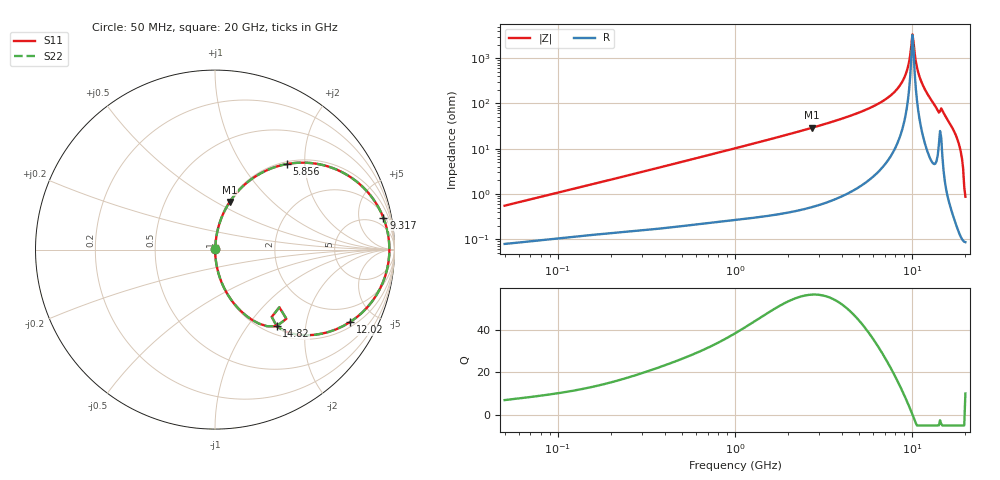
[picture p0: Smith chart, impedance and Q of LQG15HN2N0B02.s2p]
!Murata Part Number: LQG15HN2N0B02
!These Parameters are Measured in Series Mode Connection
!  o--[Z]--o
!Port1  Port2
!  o-------o
!Freq. Start=50[MHz] Stop=20[GHz], 401[Steps]
# Hz S RI R 50
!Freq.(Hz) S11(Real) S11(Imag) S21(Real) S21(Imag) S12(Real) S12(Imag) S22(Real) S22(Imag)
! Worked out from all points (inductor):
!   401 points, 50 MHz to 20 GHz, reference 50 ohm
!   read as one part in series: L = 1.72 nH near 51.52 MHz
!   highest Q = 56.5 at 2.728 GHz (marker M1), where L = 1.69 nH
!   self-resonance near 10.04 GHz
!   S11 on the Smith chart (normalised r, x): 50 MHz: 1.00, +0.01; 5.856 GHz: 1.04, +1.63; 9.317 GHz: 2, +10; 12.02 GHz: 1.21, -3.60; 14.82 GHz: 1.14, -1.39; 20 GHz: 1.00, +0.02
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5e7  0.000816 0.00544  0.9992 -0.00544  0.9992 -0.00544  0.000816 0.00544
1.364002e8  0.00139 0.0143  0.9986 -0.0143  0.9986 -0.0143  0.00139 0.0143
3.721004e8  0.00315 0.038  0.9968 -0.038  0.9968 -0.038  0.00315 0.038
1e9  0.0128 0.1002  0.9872 -0.1002  0.9872 -0.1002  0.0128 0.1002
2.728004e9  0.0817 0.2652  0.9183 -0.2652  0.9183 -0.2652  0.0817 0.2652
4.212059e9  0.1986 0.3892  0.8014 -0.3892  0.8014 -0.3892  0.1986 0.3892
5.856089e9  0.4012 0.4769  0.5988 -0.4769  0.5988 -0.4769  0.4012 0.4769
7.442007e9  0.6629 0.4516  0.3371 -0.4516  0.3371 -0.4516  0.6629 0.4516
8.516016e9  0.8415 0.3307  0.1585 -0.3307  0.1585 -0.3307  0.8415 0.3307
9.316812e9  0.938 0.1778  0.062 -0.1778  0.062 -0.1778  0.938 0.1778
9.892087e9  0.9698 0.0432  0.0302 -0.0432  0.0302 -0.0432  0.9698 0.0432
1.004137e10  0.9716 0.00642  0.0284 -0.00642  0.0284 -0.00642  0.9716 0.00642
1.034674e10  0.9666 -0.0692  0.0334 0.0692  0.0334 0.0692  0.9666 -0.0692
1.066139e10  0.949 -0.1458  0.051 0.1458  0.051 0.1458  0.949 -0.1458
1.098561e10  0.9182 -0.2204  0.0818 0.2204  0.0818 0.2204  0.9182 -0.2204
1.201863e10  0.752 -0.4039  0.248 0.4039  0.248 0.4039  0.752 -0.4039
1.375312e10  0.385 -0.4532  0.615 0.4532  0.615 0.4532  0.385 -0.4532
1.482269e10  0.3427 -0.4273  0.6573 0.4273  0.6573 0.4273  0.3427 -0.4273
1.670968e10  0.091 -0.2809  0.909 0.2809  0.909 0.2809  0.091 -0.2809
1.828096e10  0.0196 -0.1334  0.9804 0.1334  0.9804 0.1334  0.0196 -0.1334
1.88369e10  0.00839 -0.0849  0.9916 0.0849  0.9916 0.0849  0.00839 -0.0849
2e10  0.000934 0.00862  0.9991 -0.00862  0.9991 -0.00862  0.000934 0.00862
